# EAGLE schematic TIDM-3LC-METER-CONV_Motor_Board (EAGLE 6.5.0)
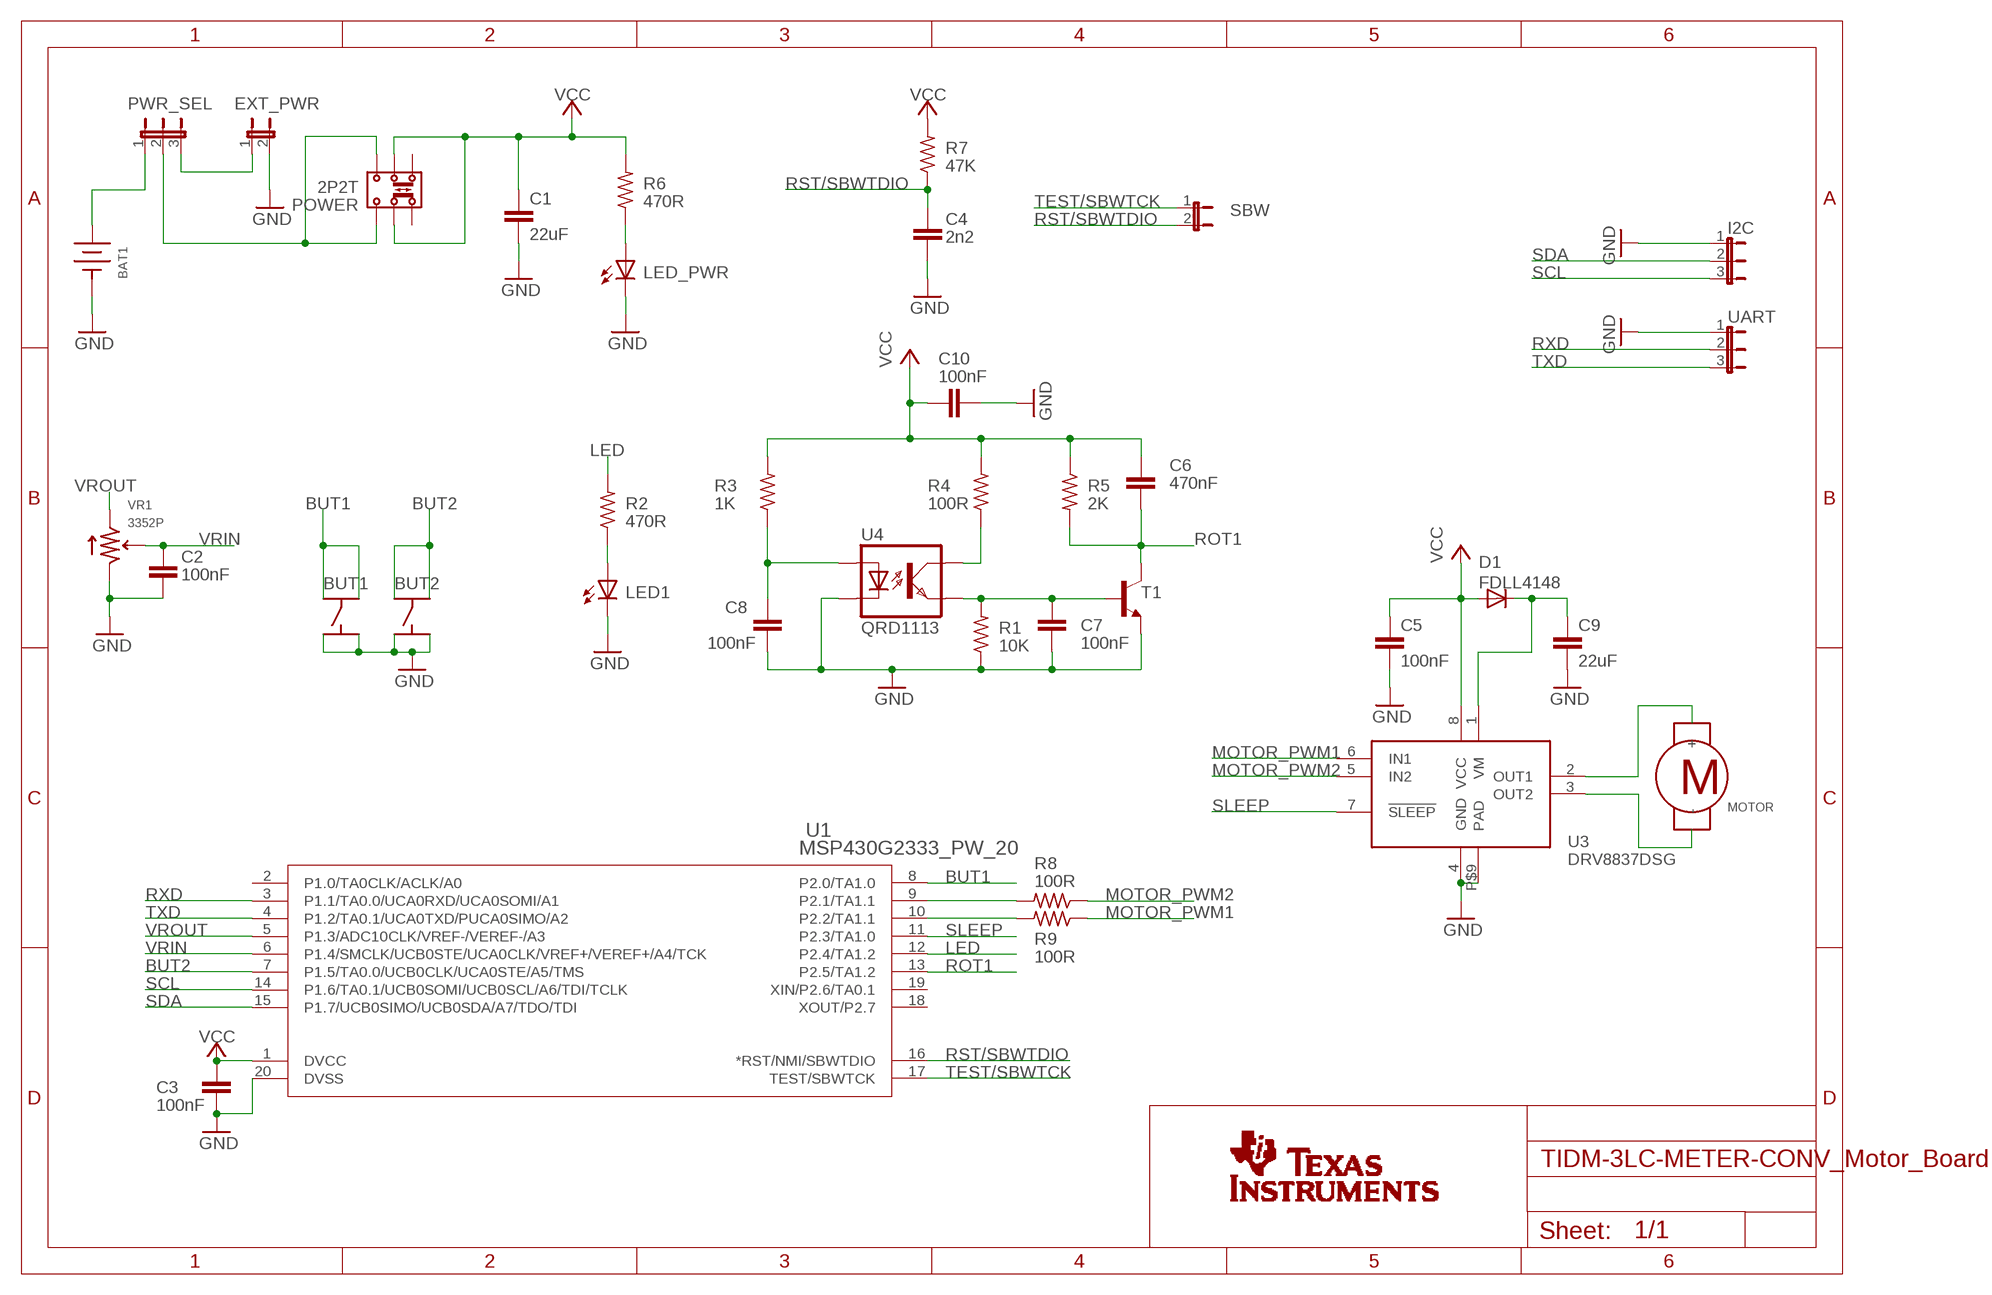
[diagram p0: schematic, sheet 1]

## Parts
BAT1  2XAAA-1  [2X3A(1_HOLE)]
BUT1  B3SL-1002P  [BUT]
BUT2  B3SL-1002P  [BUT]
C1  22uF  C-EUC1206  [C1206]
C2  100nF  C-EUC0402  [C0402]
C3  100nF  C-EUC0402  [C0402]
C4  2n2  C-EUC0402  [C0402]
C5  100nF  C-EUC0402  [C0402]
C6  470nF  C-EUC0402  [C0402]
C7  100nF  C-EUC0402  [C0402]
C8  100nF  C-EUC0402  [C0402]
C9  22uF  C-EUC1206K  [C1206K]
C10  100nF  C-EUC0402  [C0402]
D1  FDLL4148  D-SOD-80  [SOD80]
EXT_PWR  JP1E  [JP1]
I2C  JP2E  [JP2]
LED1  LEDCHIPLED_0603  [CHIPLED_0603]
LED_PWR  LEDCHIPLED_0603  [CHIPLED_0603]
MOTOR  MOTOR  [MOTOR]
POWER  2P2T  [2P2T]
PWR_SEL  JP2E  [JP2]
R1  10K  R-US_R0402  [R0402]
R2  470R  R-US_R0402  [R0402]
R3  1K  R-US_R0402  [R0402]
R4  100R  R-US_R0402  [R0402]
R5  2K  R-US_R0402  [R0402]
R6  470R  R-US_R0402  [R0402]
R7  47K  R-US_R0402  [R0402]
R8  100R  R-US_R0402  [R0402]
R9  100R  R-US_R0402  [R0402]
SBW  JP1E  [JP1]
T1  MMBT3904LT1-NPN-SOT23-BEC  [SOT23-BEC]
U1  MSP430G2333_PW_20  [PW20]
U3  DRV8837DSG  [DSG-S-PWSON-N8]
U4  QRD1113  QRD1114  [CUSTOM_4L]
U$1  TI-LOGO-SMALL  [TI-LOGO-4]
UART  JP2E  [JP2]
VR1  3352P  [3352P]

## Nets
BUT1: BUT1.P$3 BUT1.P$4 U1.8(P2.0/TA1.0)
BUT2: BUT2.P$3 BUT2.P$4 U1.7(P1.5/TA0.0/UCB0CLK/UCA0STE/A5/TMS)
GND: BAT1.- BUT1.P$1 BUT1.P$2 BUT2.P$1 BUT2.P$2 C1.2 C2.2 C3.2 C4.2 C5.2 C7.2 C8.2 C9.2 C10.2 EXT_PWR.2 I2C.1 LED1.C LED_PWR.C R1.1 T1.E U1.20(DVSS) U3.4(GND) U3.P$9(PAD) U4.P4(C) UART.1 VR1.1
LED: R2.2 U1.12(P2.4/TA1.2)
MOTOR_PWM1: R9.1 U3.6(IN1)
MOTOR_PWM2: R8.1 U3.5(IN2)
N$1: LED1.A R2.1
N$2: MOTOR.+ U3.2(OUT1)
N$3: C7.1 R1.2 T1.B U4.P2(EMIT)
N$4: MOTOR.- U3.3(OUT2)
N$5: R4.1 U4.P1(COL)
N$6: R8.2 U1.9(P2.1/TA1.1)
N$7: C9.1 D1.1(C) U3.1(VM)
N$8: R9.2 U1.10(P2.2/TA1.1)
N$10: C8.1 R3.1 U4.P3(A)
N$13: BAT1.+ PWR_SEL.1
N$14: EXT_PWR.1 PWR_SEL.3
N$15: POWER.3(3.1) POWER.6(3.2) PWR_SEL.2
N$18: LED_PWR.A R6.1
ROT1: C6.2 R5.2 T1.C U1.13(P2.5/TA1.2)
RST/SBWTDIO: C4.1 R7.1 SBW.2 U1.16(*RST/NMI/SBWTDIO)
RXD: U1.3(P1.1/TA0.0/UCA0RXD/UCA0SOMI/A1) UART.2
SCL: I2C.3 U1.14(P1.6/TA0.1/UCB0SOMI/UCB0SCL/A6/TDI/TCLK)
SDA: I2C.2 U1.15(P1.7/UCB0SIMO/UCB0SDA/A7/TDO/TDI)
SLEEP: U1.11(P2.3/TA1.0) U3.7(!SLEEP)
TEST/SBWTCK: SBW.1 U1.17(TEST/SBWTCK)
TXD: U1.4(P1.2/TA0.1/UCA0TXD/PUCA0SIMO/A2) UART.3
VCC: C1.1 C3.1 C5.1 C6.1 C10.1 D1.2(A) POWER.2(2.1) POWER.5(2.2) R3.2 R4.2 R5.1 R6.2 R7.2 U1.1(DVCC) U3.8(VCC)
VRIN: C2.1 U1.6(P1.4/SMCLK/UCB0STE/UCA0CLK/VREF+/VEREF+/A4/TCK) VR1.2
VROUT: U1.5(P1.3/ADC10CLK/VREF-/VEREF-/A3) VR1.3
Unconnected: POWER.1(1.1) POWER.4(1.2) U1.2(P1.0/TA0CLK/ACLK/A0) U1.18(XOUT/P2.7) U1.19(XIN/P2.6/TA0.1)

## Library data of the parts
BAT1 = battery:2XAAA
BUT1 BUT2 = Button:B3SL-1002P
C1-C10 = rcl:C-EU: CAPACITOR, European symbol
D1 = semicon-smd-ipc:D-: DIODE
EXT_PWR SBW = jumper:JP1E: JUMPER
I2C PWR_SEL UART = jumper:JP2E: JUMPER
LED1 LED_PWR = led:LED: LED
MOTOR = motor:MOTOR
POWER = switch:2P2T: SLIDE SWITCH 2P2T Part No. SS-22F05-G(A)4 Source: CANAL ELECTRONIC CO., LTD .. switsch.pdf
R1-R9 = rcl:R-US_: RESISTOR, American symbol
T1 = transistor:*-NPN-: NPN Transistror BF959 corrected 2008.03.06
U1 = MSP430:MSP430G2333_PW_20; DATASHEETURL: http://www.ti.com/lit/gpn/MSP430G2333; DESCRIPTION: MSP430G2x33, MSP430G2x03 Mixed Signal Microcontroller; FAMILY_NAME: Value Line; GENERIC_PART_NUMBER: MSP430G2333; INDUSTRY_STD_PKG_TYPE: TSSOP; MANUFACTURER: Texas Instruments; MANUFACTURER_PART_NUMBER: msp430g2333_pw_20; PACKAGE_DESIGNATOR: PW; PIN_COUNT: 20; VENDOR: Texas Instruments
U3 = Motor Driver:DRV8837
U4 = Opto-Sensor:QRD1114
U$1 = texas-logo:TI-LOGO: Full TI logo
VR1 = Trimmer:3352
